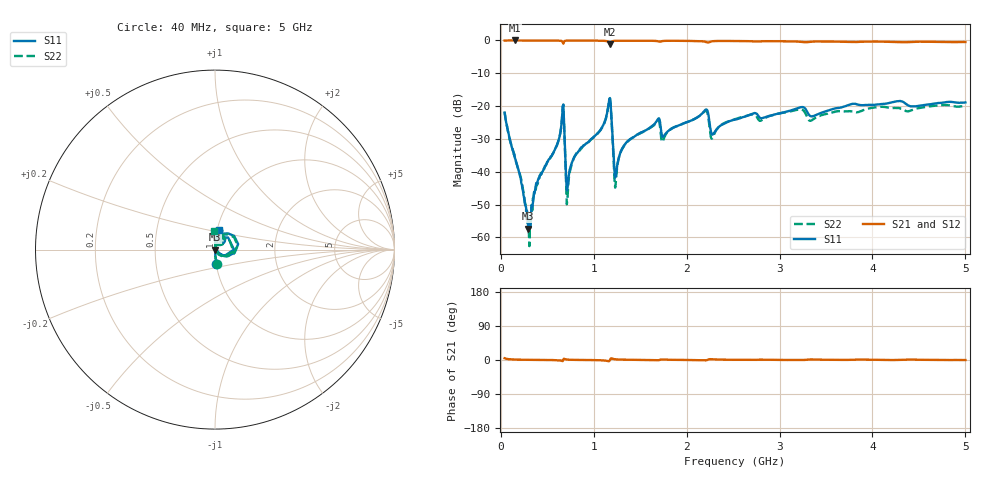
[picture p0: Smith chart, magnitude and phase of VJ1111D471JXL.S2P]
! VJ1111D471JXL
! DATE 02/15/2022  13:45
! CAPACITORS MOUNTED IN SERIES ON 25 MIL THICK MICROSTRIP SUBSTRATE
# GHz  S  MA  R  50.00
!  FREQ  S11M  S11A  S21M  S21A  S12M  S12A  S22M  S22A
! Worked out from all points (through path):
!   801 points, 40 MHz to 5 GHz, reference 50 ohm
!   highest |S21| = 0.00 dB at 151.6 MHz (marker M1); lowest = -1.2 dB at 1.175 GHz (marker M2)
!   lowest |S11| = -57.4 dB at 294.2 MHz (marker M3), VSWR 1.00, Z = 50.1 - j0.0275 ohm
!   |S11| at or under -10 dB: start of sweep to end of sweep
!   |S22| runs from -62.7 to -17.8 dB; largest |S21 - S12| = 0.011
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0.04  0.07979 -84.5  0.9963 4.6  0.9957 4.8  0.08131 -83.5
0.1516  0.01611 -84.3  0.9995 1.2  0.9958 1.3  0.01669 -86.0
0.2942  0.001351 -11.7  0.9961 0.5  0.9978 0.5  0.00181 -37.7
0.4058  0.007913 76.1  0.9953 0.2  1 0.2  0.007973 78.9
0.598  0.0244 85.1  0.9937 -0.4  0.9989 -0.5  0.0243 82.5
0.6538  0.05637 72.8  0.9806 -2.0  0.9827 -2.1  0.05589 69.1
0.6724  0.1058 0.2  0.8932 1.5  0.8955 1.4  0.1041 -5.4
0.722  0.006579 53.8  0.9939 0.9  0.9972 0.9  0.005395 63.1
0.8708  0.02379 84.5  0.9937 0.1  0.9989 0.0  0.02324 86.7
1.1746  0.1326 13.4  0.8675 0.5  0.8714 0.4  0.1282 10.1
1.218  0.01325 -23.6  0.9844 2.4  0.9887 2.3  0.01093 -32.3
1.2428  0.009955 56.2  0.9896 1.6  0.9943 1.6  0.008777 68.0
1.3544  0.02825 86.1  0.9917 0.7  0.9972 0.6  0.02792 87.7
1.6954  0.06476 71.0  0.9679 -0.5  0.9722 -0.6  0.06008 65.4
1.7512  0.03478 73.5  0.983 1.1  0.988 1.0  0.03133 81.4
2.1976  0.08665 70.0  0.9551 -1.0  0.9603 -1.1  0.08401 67.6
2.2782  0.03671 62.5  0.9719 2.0  0.9769 1.9  0.03284 72.0
2.52  0.06237 86.5  0.9796 0.5  0.9864 0.3  0.06333 90.4
3.2206  0.09539 78.6  0.9549 -0.3  0.9605 -0.5  0.08889 81.6
3.3508  0.06983 76.4  0.9592 1.4  0.964 1.2  0.06139 87.9
4.1754  0.1113 79.6  0.9525 -0.0  0.9607 -0.3  0.09443 89.8
5  0.1138 78.1  0.9467 -0.1  0.9526 -0.3  0.1017 92.8
